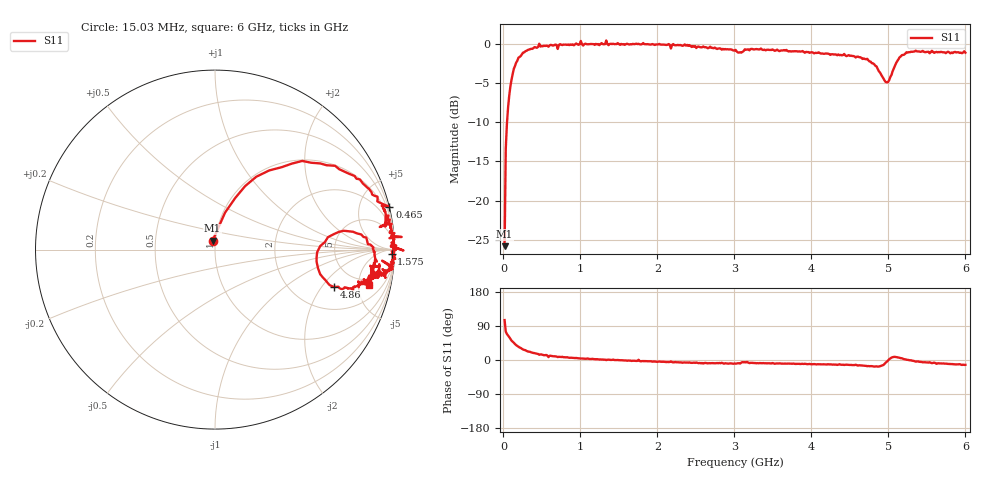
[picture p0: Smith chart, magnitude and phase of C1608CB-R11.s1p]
!	Network	Analyzer	HP8753E.07.74:	Oct	30	2002	Serial	No.	JP38451487
!	Hewlett-Packard
!	7	Sep	2009	9:54:32
!	Frequency	S11
#	HZ	S	RI	R	50
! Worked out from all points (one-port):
!   400 points, 15.03 MHz to 6 GHz, reference 50 ohm
!   lowest |S11| = -25.8 dB at 15.03 MHz (marker M1), VSWR 1.11, Z = 48.4 + j4.8 ohm
!   |S11| at or under -10 dB: start of sweep to 46.42 MHz
!   S11 on the Smith chart (normalised r, x): 15.03 MHz: 0.97, +0.10; 465 MHz: -0.02, +8.29; 1.575 GHz: 40, -59; 4.86 GHz: 3.29, -2.64; 6 GHz: 3.90, -6.64
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1.502992e7  -0.0135 0.0494
3.002985e7  0.056 0.206
6.00297e7  0.168 0.354
1.050295e8  0.371 0.459
2.550287e8  0.778 0.41
4.650277e8  0.972 0.238
5.550272e8  0.945 0.224
5.850271e8  0.949 0.128
6.150269e8  0.966 0.19
7.650262e8  0.971 0.143
1.005025e9  1.04 0.0704
1.035025e9  0.972 0.0639
1.245024e9  0.98 0.0212
1.335023e9  1.05 -0.00494
1.365023e9  0.98 0.0172
1.515022e9  0.985 -0.00964
1.575022e9  0.984 -0.0228
2.265019e9  0.978 -0.102
3.015015e9  0.902 -0.151
3.165014e9  0.915 -0.081
3.765011e9  0.882 -0.147
4.515007e9  0.819 -0.188
4.860006e9  0.662 -0.208
4.980005e9  0.566 -0.0447
5.070005e9  0.689 0.0982
5.265004e9  0.884 -0.00427
5.625002e9  0.874 -0.155
6e9  0.856 -0.195
